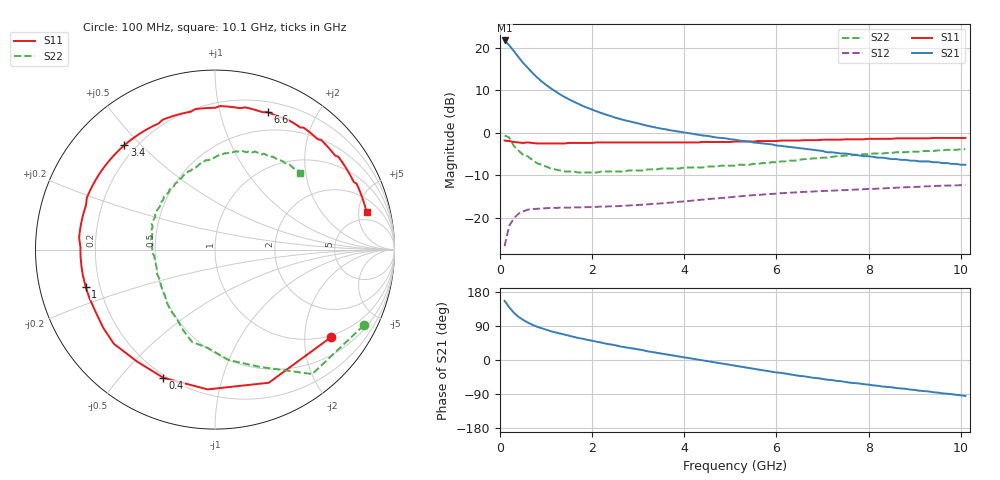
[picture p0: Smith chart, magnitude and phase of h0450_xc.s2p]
!HBFP-0450
!S and NOISE PARAMETERS at Vce=0.5V  Ic=5mA.  LAST UPDATED  09-04-98
# GHZ S MA R  50
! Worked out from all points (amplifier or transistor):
!   101 points, 100 MHz to 10.1 GHz, reference 50 ohm
!   highest |S21| = 21.8 dB at 100 MHz (marker M1)
!   |S21| within 3 dB of that: start of sweep to 335.7 MHz
!   unconditionally stable (mu >= 1): 2.928 GHz to end of sweep
!   at 1.7 GHz: K = 0.65, MSG = 12.2 dB, |S12| = -17.6 dB
!   at 5.1 GHz: K = 1.22, MAG = 3.9 dB, |S12| = -15.1 dB
!   at 10.1 GHz: K = 1.16, MAG = -0.1 dB, |S12| = -12.3 dB
!   lowest NFmin = 1.20 dB at 1.8 GHz
!   S11 on the Smith chart (normalised r, x): 100 MHz: 0.95, -2.69; 400 MHz: 0.19, -0.66; 1 GHz: 0.15, -0.14; 3.4 GHz: 0.16, +0.45; 6.6 GHz: 0.30, +1.41; 10.1 GHz: 3.54, +6.14
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0.1  0.81 -37.0  12.3 156.0  0.046 70.0  0.93 -27.0
0.2  0.8 -68.0  10.77 139.0  0.08 52.0  0.88 -52.0
0.3  0.78 -93.0  9.23 125.0  0.098 42.0  0.7 -69.0
0.4  0.77 -112.0  7.84 114.0  0.111 33.0  0.62 -83.0
0.5  0.76 -125.0  6.7 106.0  0.118 27.0  0.55 -94.0
0.6  0.77 -137.0  5.87 99.0  0.124 22.0  0.53 -104.0
0.7  0.76 -145.0  5.12 93.0  0.126 19.0  0.48 -112.0
0.8  0.75 -153.0  4.53 88.0  0.127 16.0  0.44 -119.0
1  0.75 -164.0  3.68 80.0  0.129 12.0  0.4 -132.0
1.1  0.75 -169.0  3.36 76.0  0.13 11.0  0.38 -137.0
1.2  0.75 -173.0  3.09 73.0  0.13 9.0  0.37 -142.0
1.4  0.75 179.0  2.65 67.0  0.131 7.0  0.35 -151.0
1.8  0.76 166.0  2.07 56.0  0.132 4.0  0.34 -165.0
2.1  0.77 158.0  1.79 48.0  0.134 3.0  0.34 -174.0
2.6  0.77 147.0  1.46 36.0  0.137 1.0  0.35 175.0
3.4  0.77 131.0  1.15 19.0  0.146 -2.0  0.37 160.0
3.5  0.77 129.0  1.12 17.0  0.147 -3.0  0.38 158.0
5.1  0.79 98.0  0.83 -15.0  0.176 -14.0  0.41 129.0
6.6  0.82 69.0  0.65 -43.0  0.201 -30.0  0.49 99.0
6.8  0.82 65.0  0.63 -47.0  0.203 -32.0  0.5 96.0
8.5  0.85 38.0  0.49 -72.0  0.224 -51.0  0.58 69.0
10.1  0.87 14.0  0.42 -95.0  0.242 -72.0  0.64 42.0
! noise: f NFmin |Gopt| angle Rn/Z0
1.8  1.2  0.6  168  0.03
2  1.26  0.59  177  0.03
2.5  1.45  0.61  -168  0.05
3.5  1.76  0.69  -142  0.16
4  1.99  0.7  -129  0.31
5  2.3  0.75  -106  0.73
5.5  2.54  0.78  -95  1.09
7  2.97  0.83  -64  2.5
8  3.34  0.82  -48  3.57
10  3.95  0.81  -17  5.83
